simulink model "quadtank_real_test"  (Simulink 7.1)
settings: Solver=ode45  StartTime=0.0  StopTime=inf  RelTol=1e-3
libraries: simulink x2, tank x1

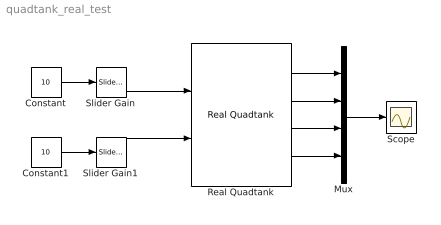
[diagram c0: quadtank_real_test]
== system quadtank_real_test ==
  Constant : Constant  Value=10  OutDataType=sfix(16)  OutScaling=2^0
  Constant1 : Constant  Value=10  OutDataType=sfix(16)  OutScaling=2^0
  Mux : Mux
  Real Quadtank : tank/Real Quadtank  SystemSampleTime=-1  h=0.05
  Scope : Scope
  Slider Gain : simulink/Math Operations/Slider Gain  SystemSampleTime=-1  low=0  gain=0  high=1
  Slider Gain1 : simulink/Math Operations/Slider Gain  SystemSampleTime=-1  low=0  gain=0  high=1
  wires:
  Slider Gain/1 -> Real Quadtank/1
  Slider Gain1/1 -> Real Quadtank/2
  Constant/1 -> Slider Gain/1
  Constant1/1 -> Slider Gain1/1
  Real Quadtank/4 -> Mux/4
  Real Quadtank/3 -> Mux/3
  Real Quadtank/2 -> Mux/2
  Real Quadtank/1 -> Mux/1
  Mux/1 -> Scope/1
